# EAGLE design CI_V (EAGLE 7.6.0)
DATABASE: /Users/Kevin/working/CAD_Parts/IHC_Parts_DB.txt

## Sheet 1 of 4: CI-V Arduino Shield
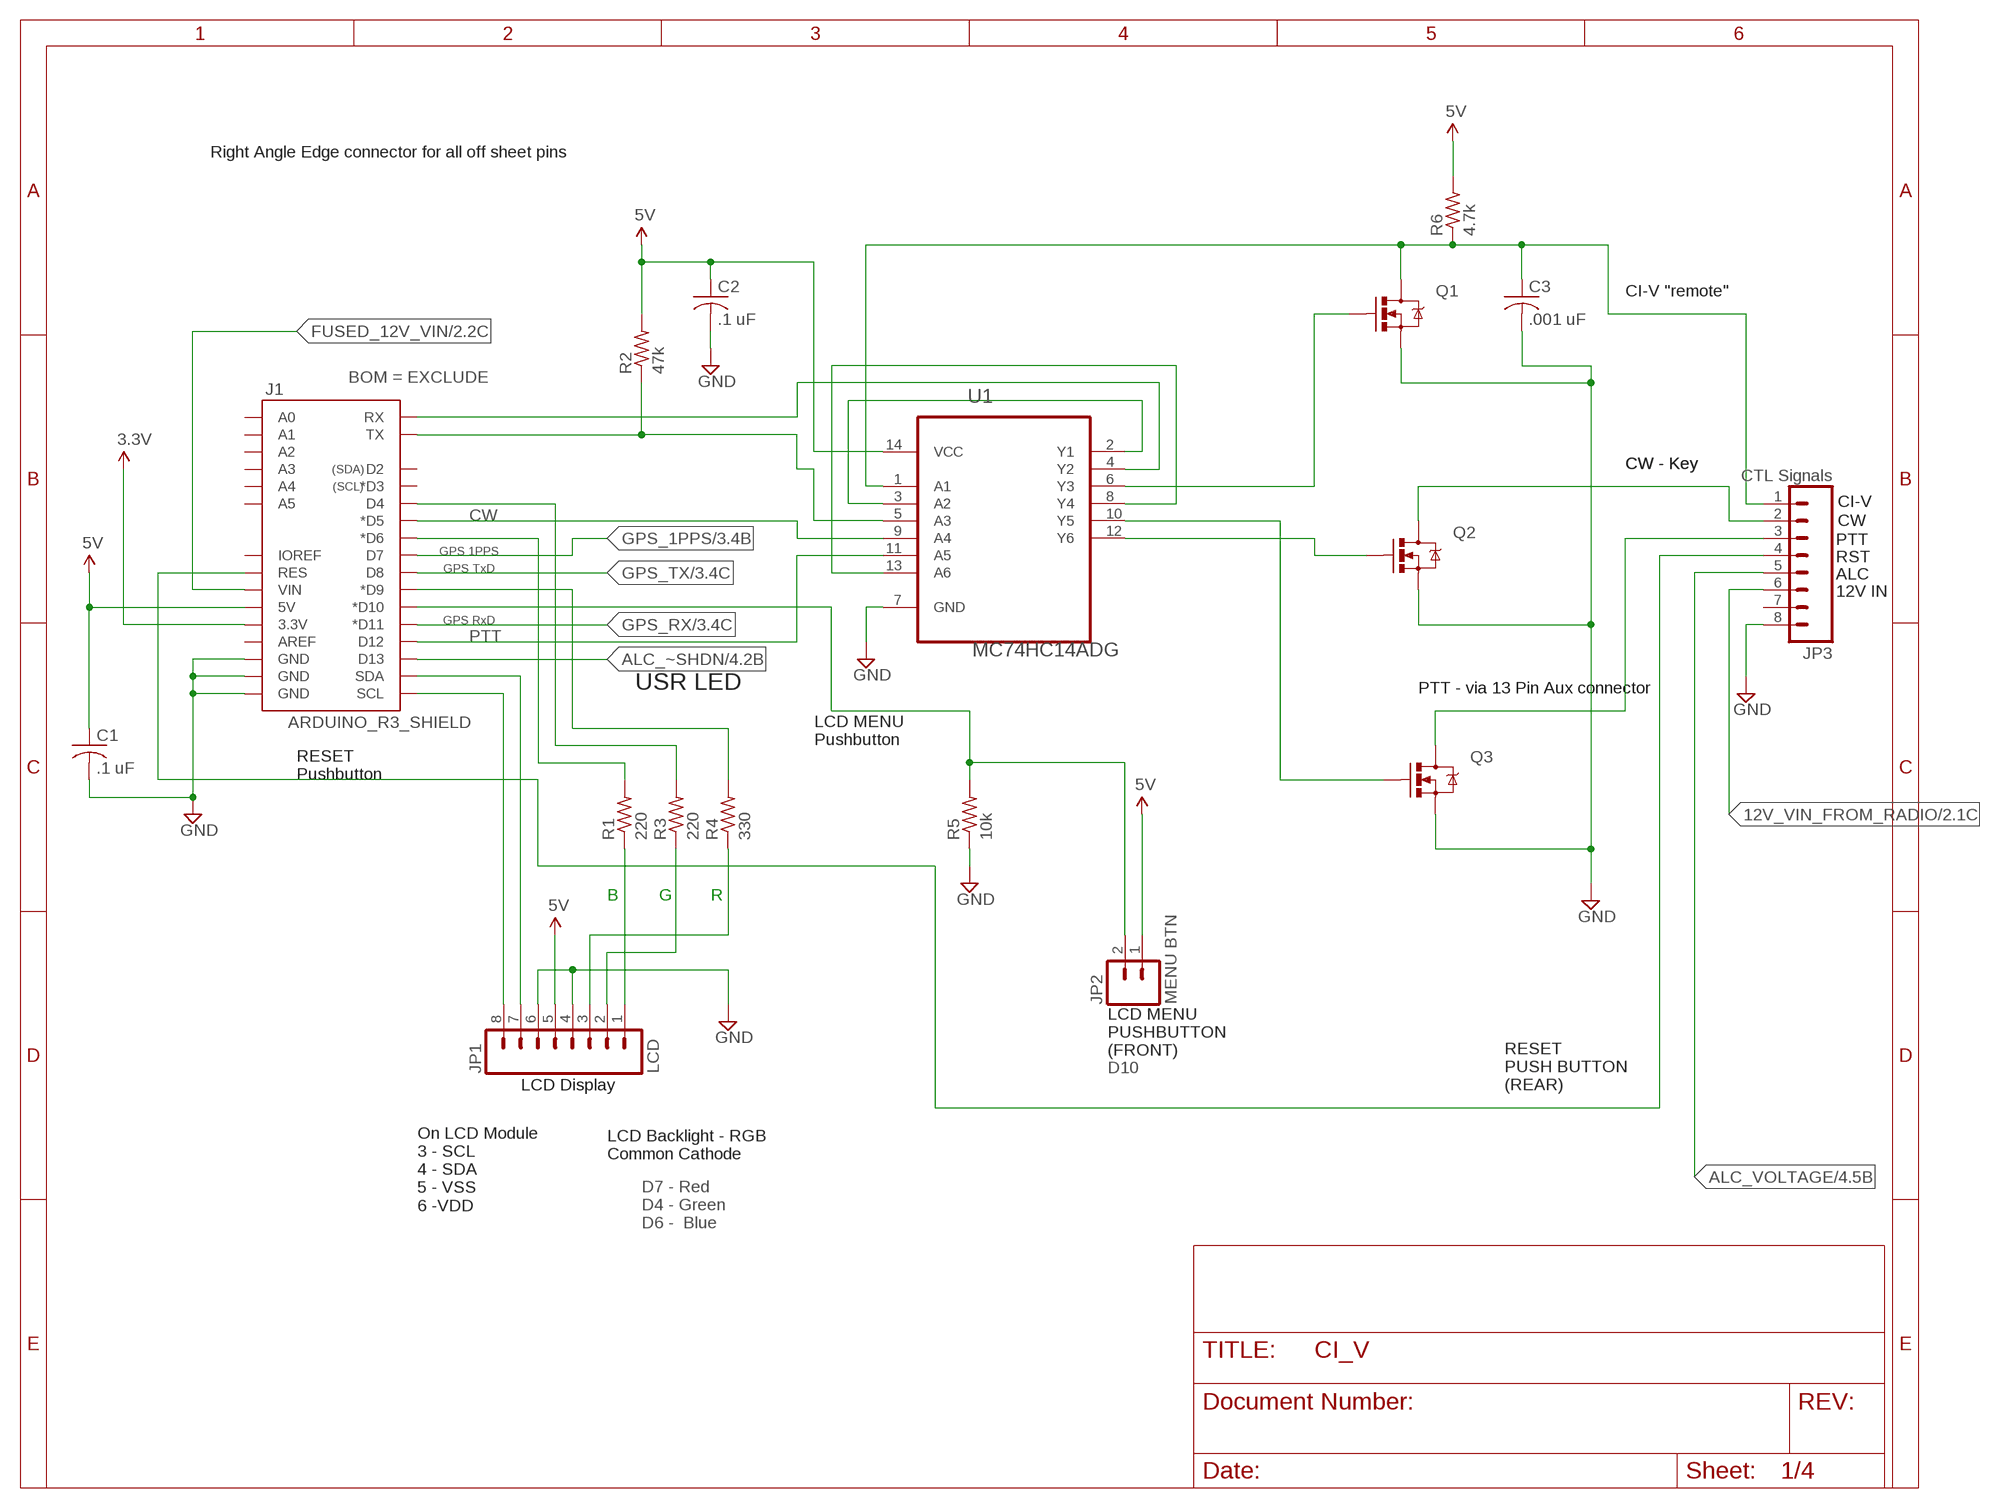
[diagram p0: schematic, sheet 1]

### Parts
C1  .1 uF  C-USC0805  [C0805]
C2  .1 uF  C-USC0805  [C0805]
C3  .001 uF  C-USC0805  [C0805]
J1  ARDUINO_R3_SHIELD  [UNO_R3_SHIELD]
JP1  LCD  M08NO_SILK  [1X08_PIN1_NO_SILK]
JP2  MENU BTN  M02PTH  [1X02]
JP3  CTL Signals  M08NO_SILK  [1X08_PIN1_NO_SILK]
Q1  MOSFET-NCHANNELBSS123LT1G  [SOT23-3]
Q2  MOSFET-NCHANNELBSS123LT1G  [SOT23-3]
Q3  MOSFET-NCHANNELBSS123LT1G  [SOT23-3]
R1  220  R-US_R0805  [R0805]
R2  47k  R-US_R0805  [R0805]
R3  220  R-US_R0805  [R0805]
R4  330  R-US_R0805  [R0805]
R5  10k  R-US_R0805  [R0805]
R6  4.7k  R-US_R0805  [R0805]
U1  MC74HC14ADG  [SOIC127P600X175-14N]

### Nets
3.3V: J1.3.3V ; also sheet 3
5V: C1.1 C2.1 J1.5V JP1.5 JP2.1 R2.2 R6.2 U1.14(VCC) ; also sheet 4
12V_VIN_FROM_RADIO: JP3.6 ; also sheet 2
ALC_VOLTAGE: JP3.5 ; also sheet 4
ALC_~SHDN: J1.D13 ; also sheet 4
CW: J1.D5(*D5) U1.9(A4)
FUSED_12V_VIN: J1.VIN ; also sheet 2
GND: C1.2 C2.2 C3.2 J1.GND@0(GND) J1.GND@1(GND) J1.GND@2(GND) JP1.4 JP1.6 JP3.8 Q1.2(S) Q2.2(S) Q3.2(S) R5.1 U1.7(GND) ; also sheet 2,3,4
GPS_1PPS: J1.D7 ; also sheet 3
GPS_RX: J1.D11(*D11) ; also sheet 3
GPS_TX: J1.D8 ; also sheet 3
HARD_RX: J1.RX U1.4(Y2)
HARD_TX: J1.TX R2.1 U1.5(A3)
N$1: C3.1 JP3.1 Q1.3(D) R6.1 U1.1(A1)
N$2: JP3.2 Q2.3(D)
N$3: JP3.3 Q3.3(D)
N$4: Q1.1(G) U1.6(Y3)
N$5: JP1.1 R1.1
N$7: JP1.2 R3.1
N$8: U1.2(Y1) U1.3(A2)
N$9: Q2.1(G) U1.12(Y6)
N$10: Q3.1(G) U1.10(Y5)
N$12: J1.SCL JP1.8
N$13: U1.8(Y4) U1.13(A6)
N$14: J1.SDA JP1.7
N$15: JP1.3 R4.1
N$16: J1.D6(*D6) R1.2
N$17: J1.D4 R3.2
N$18: J1.D9(*D9) R4.2
N$19: J1.D10(*D10) JP2.2 R5.2
N$20: J1.RES JP3.4
PTT: J1.D12 U1.11(A5)
Unconnected: J1.A0 J1.A1 J1.A2 J1.A3 J1.A4 J1.A5 J1.AREF J1.D2 J1.D3(*D3) J1.IOREF JP3.7

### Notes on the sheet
- Right Angle Edge connector for all off sheet pins
- CI-V "remote"
- CW - Key | CW - Key
- CI-V
- CW
- PTT
- GPS 1PPS
- RST
- GPS TxD
- ALC
- 12V IN
- GPS RxD
- USR LED | PTT - via 13 Pin Aux connector
- LCD MENU
  Pushbutton
- RESET
  Pushbutton
- B | G | R
- LCD MENU
  PUSHBUTTON
  (FRONT)
- D10
- LCD Display
- RESET
  PUSH BUTTON
  (REAR)
- LCD Backlight - RGB
  Common Cathode
- On LCD Module
  3 - SCL
  4 - SDA
  5 - VSS
  6 -VDD
- D7 - Red
  D4 - Green
  D6 -  Blue

## Sheet 2 of 4: Power
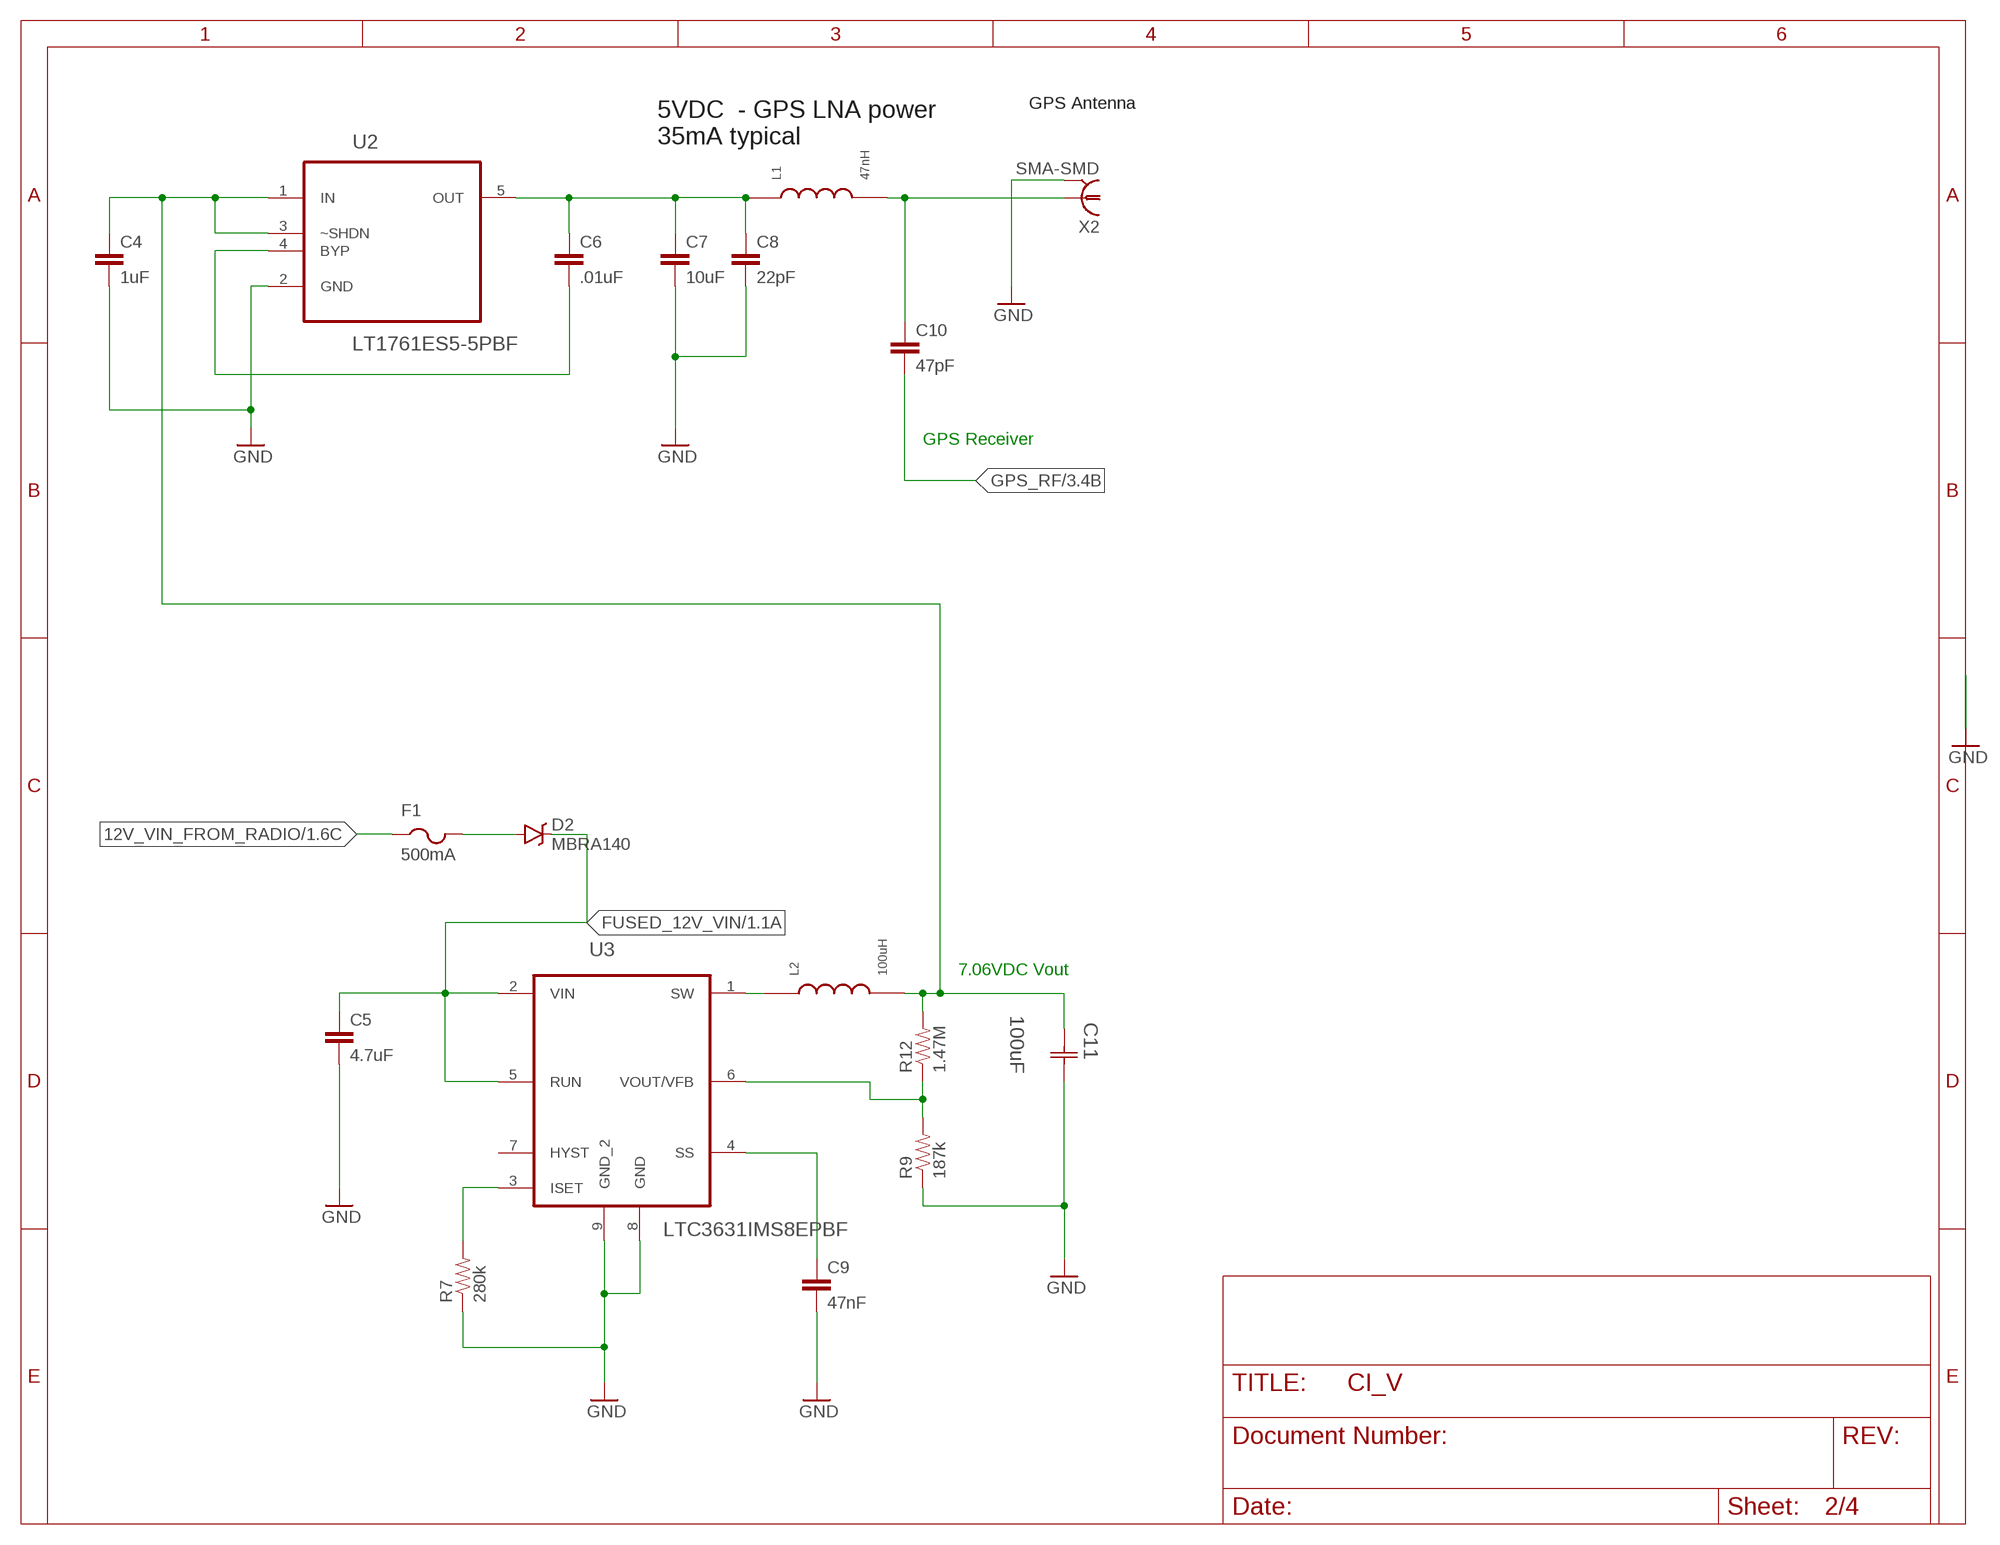
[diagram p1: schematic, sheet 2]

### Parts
C4  1uF  CAP0805  [0805]
C5  4.7uF  CAP1210  [1210]
C6  .01uF  CAP0805  [0805]
C7  10uF  CAP1210  [1210]
C8  22pF  CAP0805  [0805]
C9  47nF  CAP0805  [0805]
C10  47pF  CAP0805  [0805]
C11  100uF  THJC226K016RJN  [CAPCP6032X280N]
D2  MBRA140  DIODE-SCHOTTKY-MBRA140  [SMA-DIODE]
F1  500mA  PTCFUSE-1206  [R1206]
L1  47nH  INDUCTORMURATA  [0805]
L2  100uH  INDUCTORMURATATDK  [SLF7045]
R7  280k  RESISTOR0805-RES  [0805]
R9  187k  RESISTOR0805-RES  [0805]
R12  1.47M  RESISTOR0805-RES  [0805]
U2  LT1761ES5-5PBF  [SOT95P280X100-5N]
U3  LTC3631IMS8EPBF  [SOP65P490X110-9N]
X2  SMA-SMD  [SMA-SMD]

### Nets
7V_BUS: C4.1 C11.1(C1) L2.2 R12.2 U2.1(IN) U2.3(~SHDN)
12V_VIN_FROM_RADIO: F1.1 ; also sheet 1
FUSED_12V_VIN: C5.1 D2.C U3.2(VIN) U3.5(RUN) ; also sheet 1
GND: C4.2 C5.2 C7.2 C8.2 C9.2 C11.2(C2) R7.1 R9.1 U2.2(GND) U3.8(GND) U3.9(GND_2) X2.2@1 X2.2@2 X2.2@3 X2.2@4 X2.2@5 X2.2@6 ; also sheet 1,3,4
GPS_RF: C10.2 ; also sheet 3
ISET: R7.2 U3.3(ISET)
N$6: C10.1 L1.2 X2.1
N$21: C6.2 U2.4(BYP)
N$25: D2.A F1.2
SS: C9.1 U3.4(SS)
SW: L2.1 U3.1(SW)
VCC: C6.1 C7.1 C8.1 L1.1 U2.5(OUT)
VFB: R9.2 R12.1 U3.6(VOUT/VFB)
Unconnected: U3.7(HYST)

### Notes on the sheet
- GPS Antenna
- 5VDC  - GPS LNA power
  35mA typical
- GPS Receiver
- 7.06VDC Vout

## Sheet 3 of 4: GPS Receiver
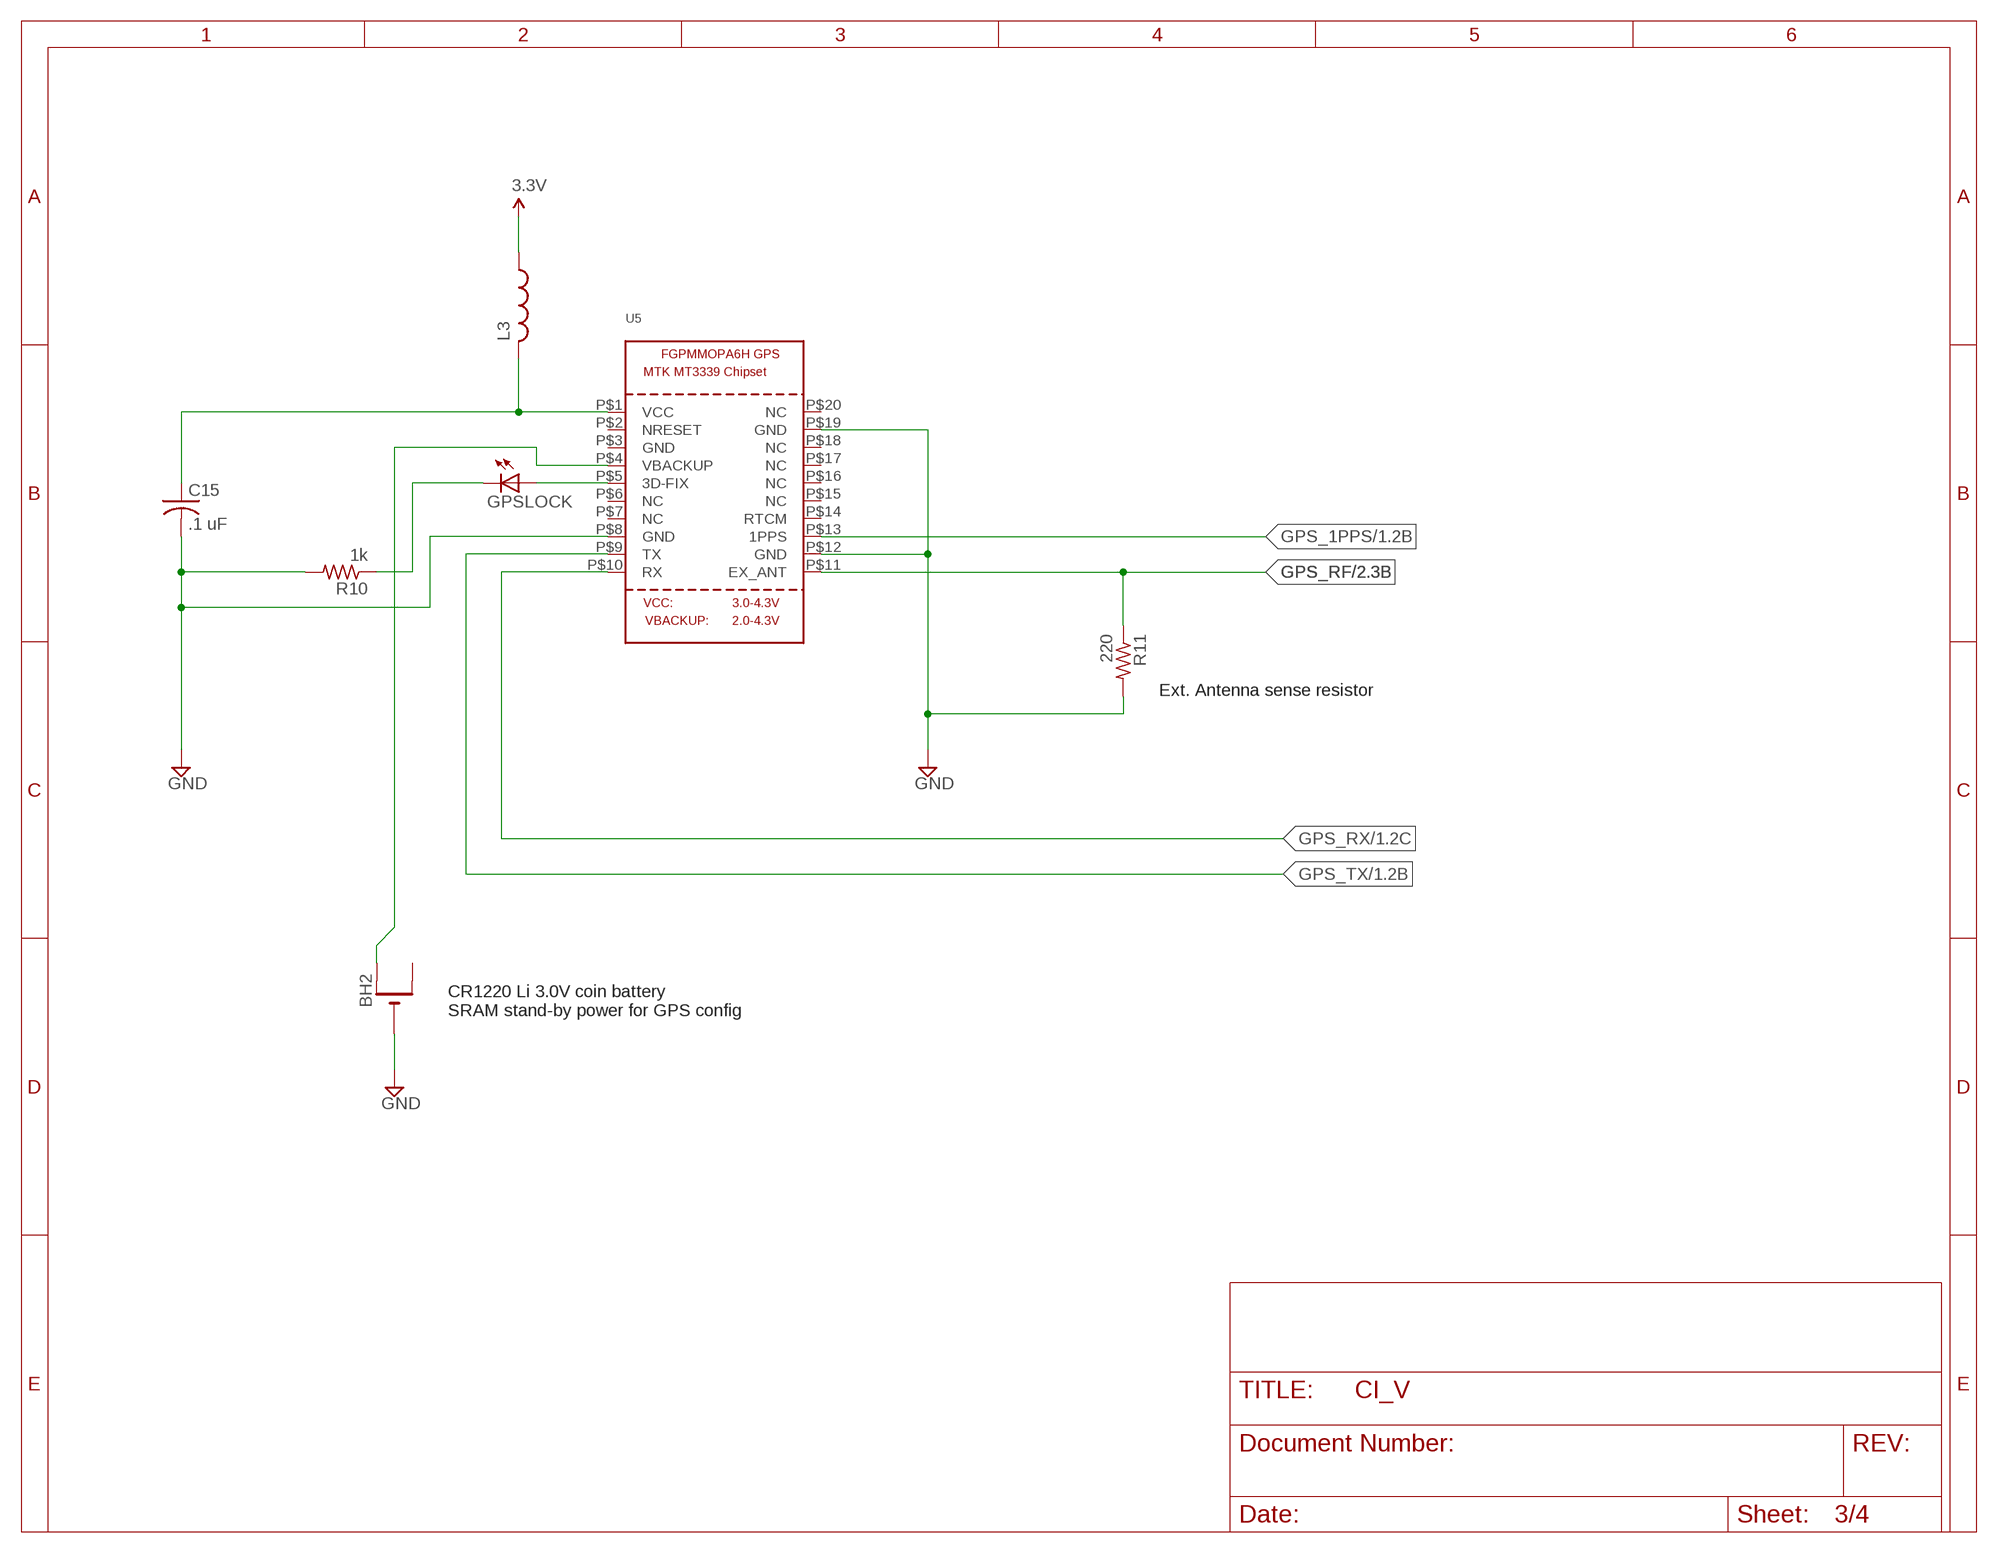
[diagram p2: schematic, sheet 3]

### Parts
BH2  CR1220SMT  [CR1220-SMD]
C15  .1 uF  C-USC0805  [C0805]
GPSLOCK  LEDCHIPLED_0805  [CHIPLED_0805]
L3  L-USL2012C  [L2012C]
R10  1k  R-US_R0805  [R0805]
R11  220  R-US_R0805  [R0805]
U5  GPS_FGPMMOPA6H  [FGPMMOPA6H]

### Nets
3.3V: L3.1 ; also sheet 1
GND: BH2.- C15.2 R10.2 R11.2 U5.P$8(GND) U5.P$12(GND) U5.P$19(GND) ; also sheet 1,2,4
GPS_1PPS: U5.P$13(1PPS) ; also sheet 1
GPS_BATT: BH2.+$1(+) U5.P$4(VBACKUP)
GPS_RF: R11.1 U5.P$11(EX_ANT) ; also sheet 2
GPS_RX: U5.P$10(RX) ; also sheet 1
GPS_TX: U5.P$9(TX) ; also sheet 1
N$11: C15.1 L3.2 U5.P$1(VCC)
N$22: GPSLOCK.A U5.P$5(3D-FIX)
N$23: GPSLOCK.C R10.1
Unconnected: BH2.+$2(+1) U5.P$2(NRESET) U5.P$3(GND) U5.P$6(NC) U5.P$7(NC) U5.P$14(RTCM) U5.P$15(NC) U5.P$16(NC) U5.P$17(NC) U5.P$18(NC) U5.P$20(NC)

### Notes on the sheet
- Ext. Antenna sense resistor
- CR1220 Li 3.0V coin battery
  SRAM stand-by power for GPS config

## Sheet 4 of 4: ALC control
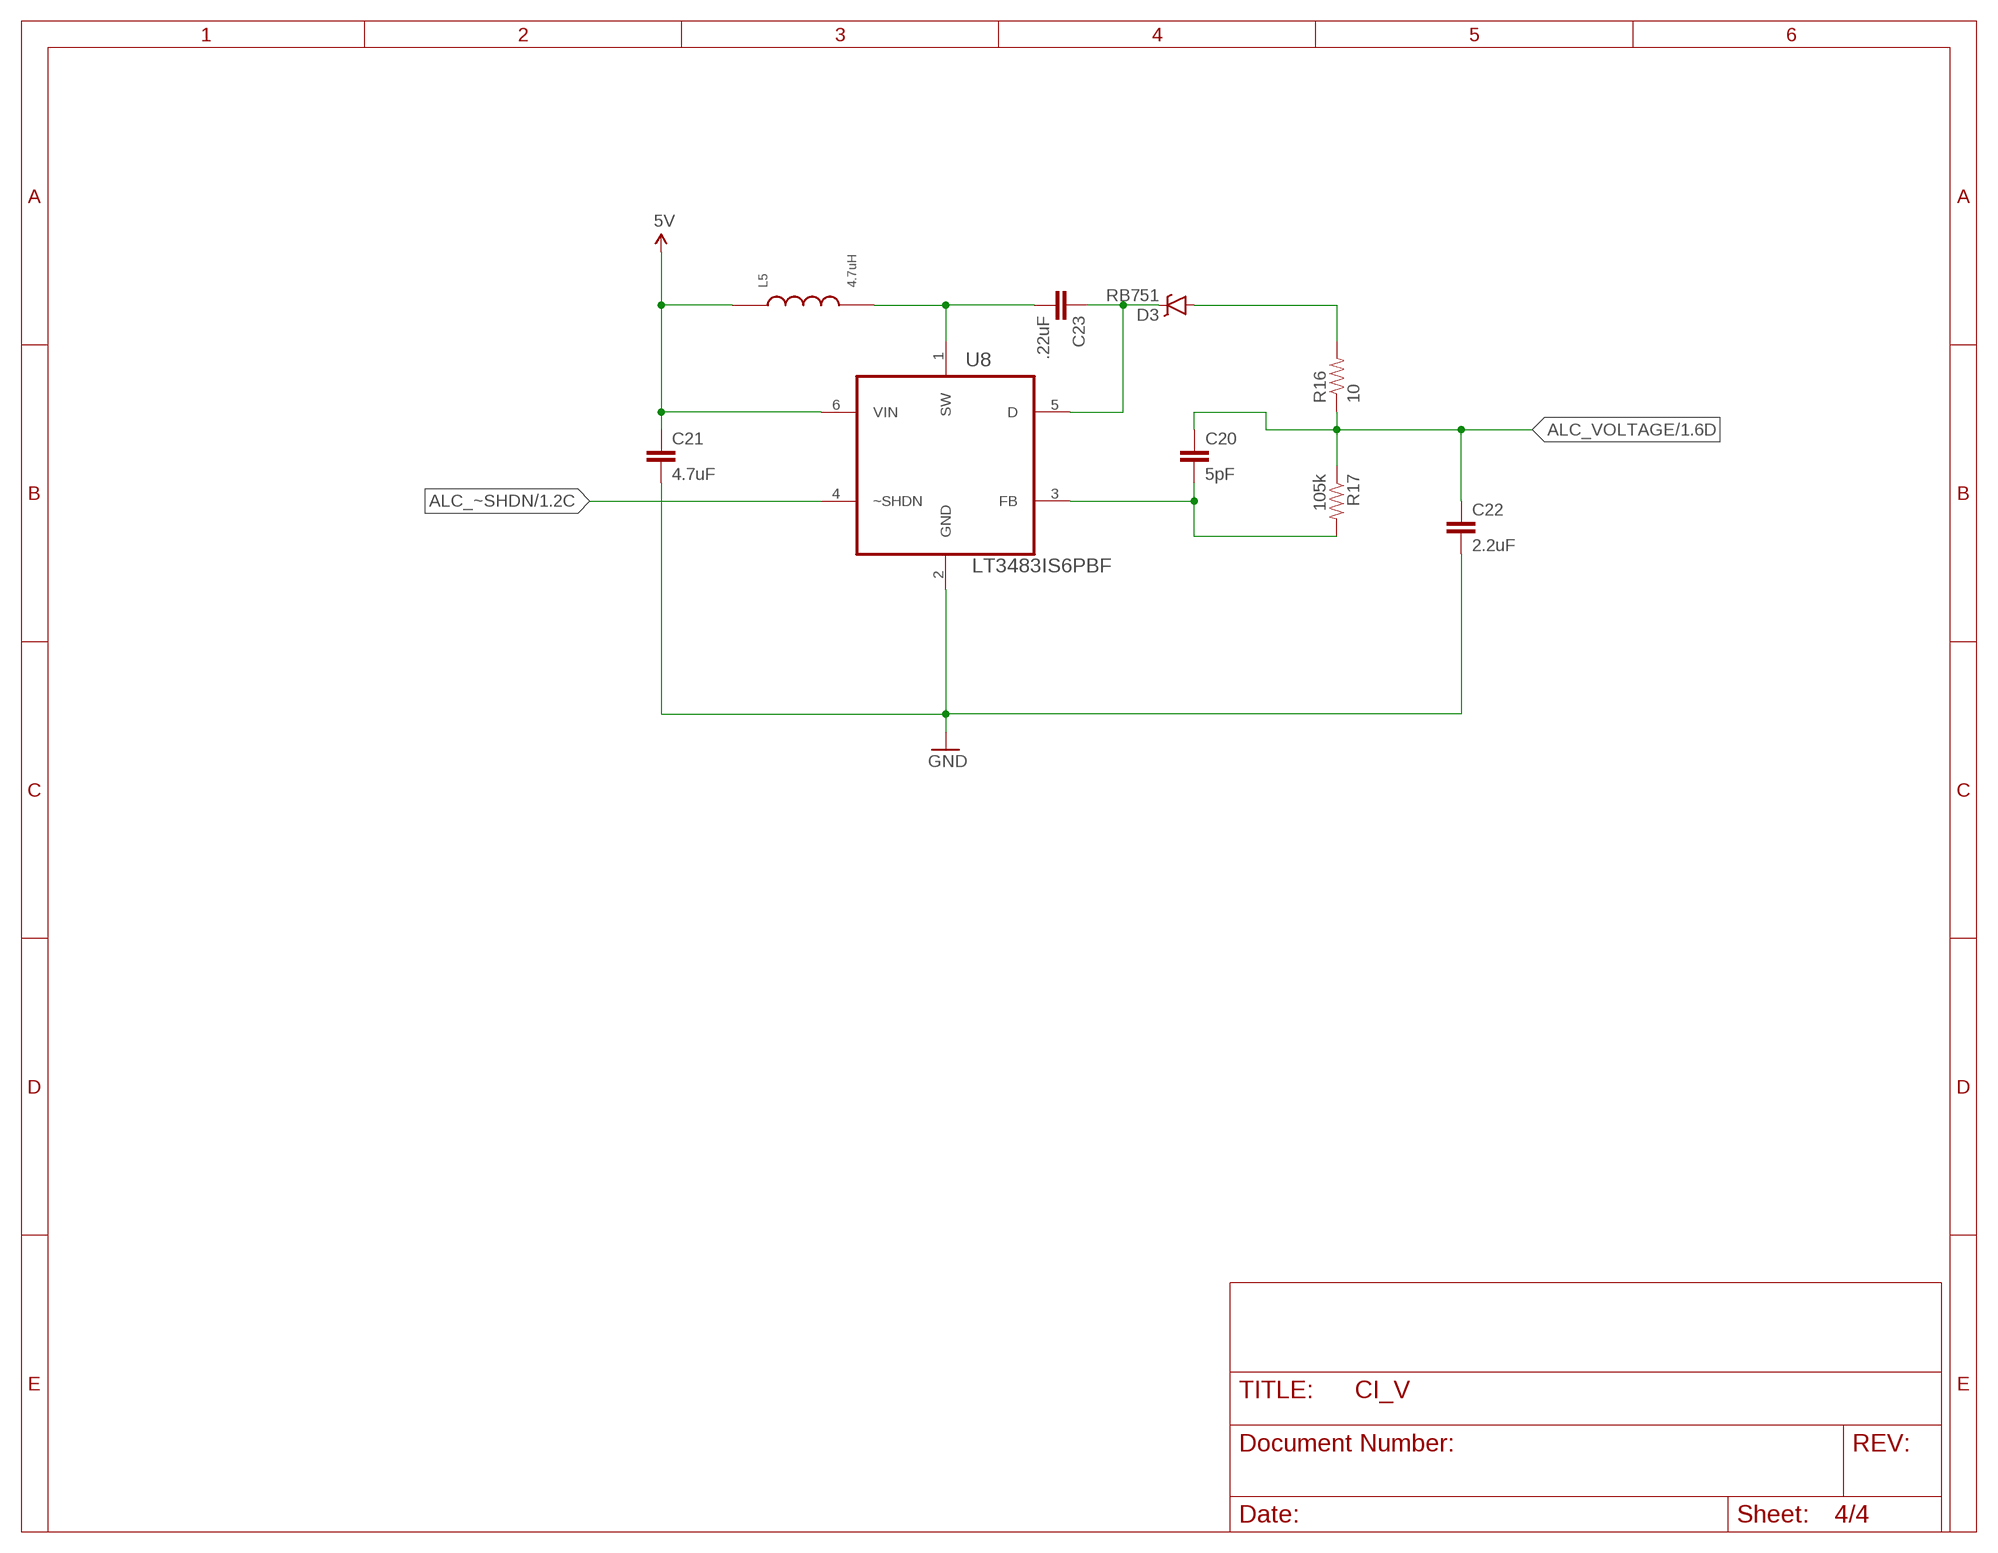
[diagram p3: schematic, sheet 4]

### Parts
C20  5pF  CAP0805  [0805]
C21  4.7uF  CAP1210  [1210]
C22  2.2uF  CAP0805  [0805]
C23  .22uF  CAP0805  [0805]
D3  RB751  DIODE-SCHOTTKY-RB751  [SOD-523]
L5  4.7uH  INDUCTORMURATA  [0805]
R16  10  RESISTOR0805-RES  [0805]
R17  105k  RESISTOR0805-RES  [0805]
U8  LT3483IS6PBF  [SOT95P280X100-6N]

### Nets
5V: C21.1 L5.1 U8.6(VIN) ; also sheet 1
ALC_VOLTAGE: C20.1 C22.1 R16.1 R17.1 ; also sheet 1
ALC_~SHDN: U8.4(~SHDN) ; also sheet 1
GND: C21.2 C22.2 U8.2(GND) ; also sheet 1,2,3
N$28: C23.2 L5.2 U8.1(SW)
N$33: C23.1 D3.C U8.5(D)
N$34: D3.A R16.2
N$37: C20.2 R17.2 U8.3(FB)

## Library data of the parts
BH2 = IHC:CR1220: CR1216/CR1220/CR1225 12mm 3V lithium coin cell Great for battery packup. Both SMT and THM holders. Note the THM package has the ground pads on both sides of the PCB so that the masks are the same - this reduces the cost; PARTNO: 165-0001-001
C1 C2 C15 = rcl:C-US: CAPACITOR, American symbol; PARTNO: 120-0001-010
C3 = rcl:C-US: CAPACITOR, American symbol; PARTNO: 120-0001-015
C4 = SparkFun-Capacitors:CAP: Capacitor; PARTNO: 120-0001-015
C5 C21 = SparkFun-Capacitors:CAP: Capacitor; PARTNO: 120-0003-011
C6 = SparkFun-Capacitors:CAP: Capacitor; PARTNO: 120-0001-020
C7 = SparkFun-Capacitors:CAP: Capacitor; PARTNO: 120-0003-010
C8 = SparkFun-Capacitors:CAP: Capacitor; PARTNO: 120-0004-011
C9 = SparkFun-Capacitors:CAP: Capacitor; PARTNO: 120-0001-013
C10 C20 = SparkFun-Capacitors:CAP: Capacitor; PARTNO: 120-0004-010
C11 = AVX_By_element14_Batch_1:THJC226K016RJN: Tantalum Capacitor , 2312; CAPACITANCETOLERANCE: ±10%; MPN: THJC226K016RJN; OC_FARNELL: 1707045; OC_NEWARK: 57P7383; PARTNO: 120-0005-050; SUPPLIER: AVX; VALUE: 22µF; VOLTAGERATING: 16V
C22 = SparkFun-Capacitors:CAP: Capacitor; PARTNO: 120-0002-011
C23 = SparkFun-Capacitors:CAP: Capacitor; PARTNO: 120-0001-022
D2 = SparkFun-DiscreteSemi:DIODE-SCHOTTKY: Schottky diodes in SFE's production catalog; PARTNO: 140-0001-001; PROD_ID: DIO-08053
D3 = SparkFun-DiscreteSemi:DIODE-SCHOTTKY: Schottky diodes in SFE's production catalog; PARTNO: 140-0002-001; PROD_ID: DIO-11018
F1 = adafruit:PTCFUSE: PTC fuses, resettable thermistors; PARTNO: 145-0001-001
GPSLOCK = adafruit:LED: LED; PARTNO: 160-0007-001
J1 = IHC:ARDUINO_R3_SHIELD: Shield form compatible with the Arduino Uno R3.; BOM: EXCLUDE
JP1 JP3 = SparkFun-Connectors:M08: Header 8 Standard 8-pin 0.1" header. Use with straight break away headers (SKU : PRT-00116), right angle break away headers (PRT-00553), swiss pins (PRT-00743), machine pins (PRT-00117), and female headers (PRT-00115).; PARTNO: 125-0019-001
JP2 = IHC:M02: Standard 2-pin 0.1" header. Use with; PARTNO: 125-0019-001
L1 = IHC:INDUCTOR; PARTNO: 155-0002-001
L2 = IHC:INDUCTOR; PARTNO: 155-0001-001
L3 = rcl:L-US: INDUCTOR, American symbol; PARTNO: 155-0004-001
L5 = IHC:INDUCTOR; PARTNO: 155-0003-001
Q1-Q3 = SparkFun-DiscreteSemi:MOSFET-NCHANNEL: Common NMOSFET Parts MFG P/NStore IDProd ID FDD8780TRANS-09984 SI7820DNTRANS-11055 FDS6630AIC-08089 2N7002PWTRANS-11151 FQP30N06L COM-10213TRANS-10060 BSS123LT1GTRANS-08345 BSS138TRANS-00830 BS170 2N7000; PARTNO: 185-0001-001; PROD_ID: TRANS-08345
R1 R3 R11 = rcl:R-US_: RESISTOR, American symbol; PARTNO: 110-0001-010
R2 R6 = rcl:R-US_: RESISTOR, American symbol; PARTNO: 110-0001-030
R4 R5 = rcl:R-US_: RESISTOR, American symbol; PARTNO: 110-0001-025
R7 = SparkFun-Passives:RESISTOR: Resistor; PARTNO: 110-0002-015
R9 = SparkFun-Passives:RESISTOR: Resistor; PARTNO: 110-0002-020
R10 = rcl:R-US_: RESISTOR, American symbol; PARTNO: 110-0001-029
R12 = SparkFun-Passives:RESISTOR: Resistor; PARTNO: 110-0002-010
R16 = SparkFun-Passives:RESISTOR: Resistor; PARTNO: 110-0001-027
R17 = SparkFun-Passives:RESISTOR: Resistor; PARTNO: 110-0003-010
U1 = ON Semiconductor_By_element14_Batch_1:MC74HC14ADG: Hex Schmitt-Trigger Inverter; MPN: MC74HC14ADG; OC_FARNELL: 9666931; OC_NEWARK: 71J5595; PACKAGE: SOIC-14; PARTNO: 200-0001-001; SUPPLIER: ON SEMICONDUCTOR
U2 = LTC_By_element14_Batch_1:LT1761ES5-5PBF: 100mA, Low Noise,LDO Micropower Regulators; MPN: LT1761ES5-5#PBF; OC_FARNELL: 1533302; OC_NEWARK: 61M3359; PACKAGE: TSOT-23-5; PARTNO: 230-0002-001; SUPPLIER: Linear Technology
U3 = IHC:LTC3631IMS8EPBF: Step-Down Converter; MPN: LTC3631IMS8E#PBF; OC_FARNELL: -; OC_NEWARK: 24R8687; PACKAGE: MSOP-8; PARTNO: 230-0003-001; SUPPLIER: Linear Technology
U5 = adafruit:GPS_FGPMMOPA6H: GPS Module - MTK MT3339 Chipset, -165dBm sensitivity, 22 channels, 10Hz, auto-select external antenna options; PARTNO: 240-0001-001
U8 = IHC:LT3483IS6PBF: Inverting Micropower DC/DC Converters with Schottky; MPN: LT3483IS6#PBF; OC_FARNELL: -; OC_NEWARK: 84R9683; PACKAGE: TSOT-23-6; SUPPLIER: Linear Technology
X2 = con-coax:SMA-SMD: SMA 50 Ohm Straight Jack Receptacle - Surface Mount; OC_FARNELL: unknown; OC_NEWARK: unknown; PARTNO: 125-0018-001

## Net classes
0 default: clearance 0.205 mm

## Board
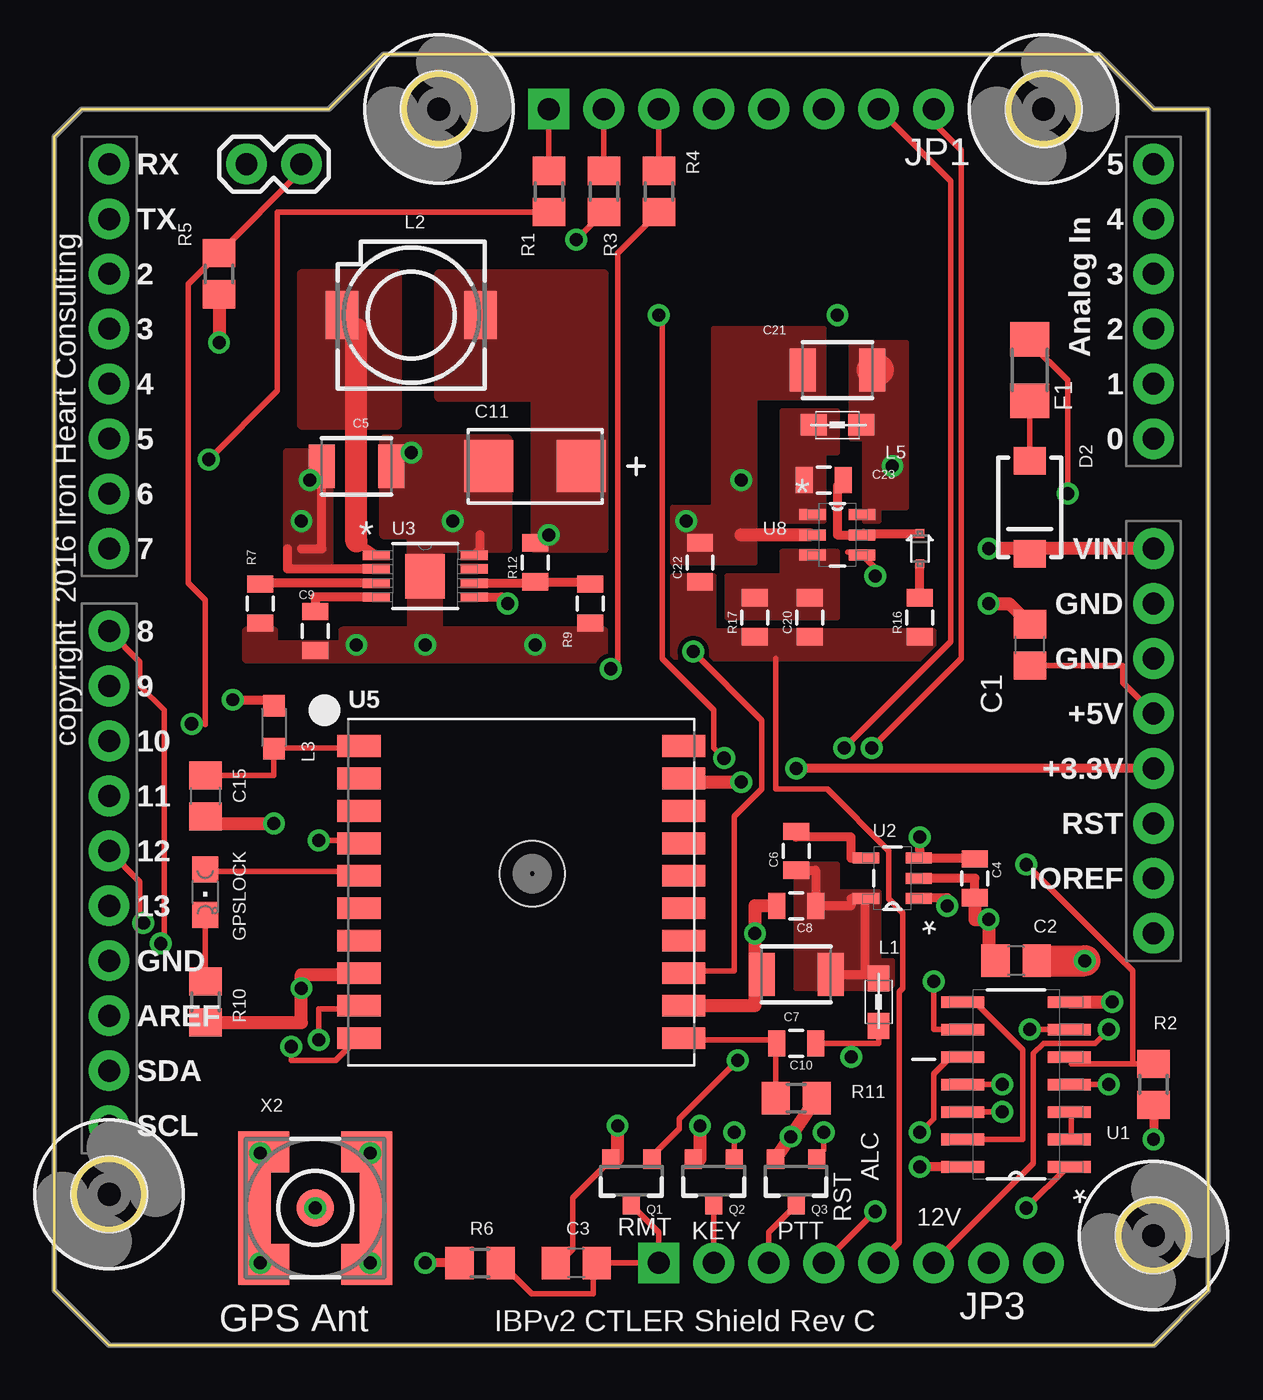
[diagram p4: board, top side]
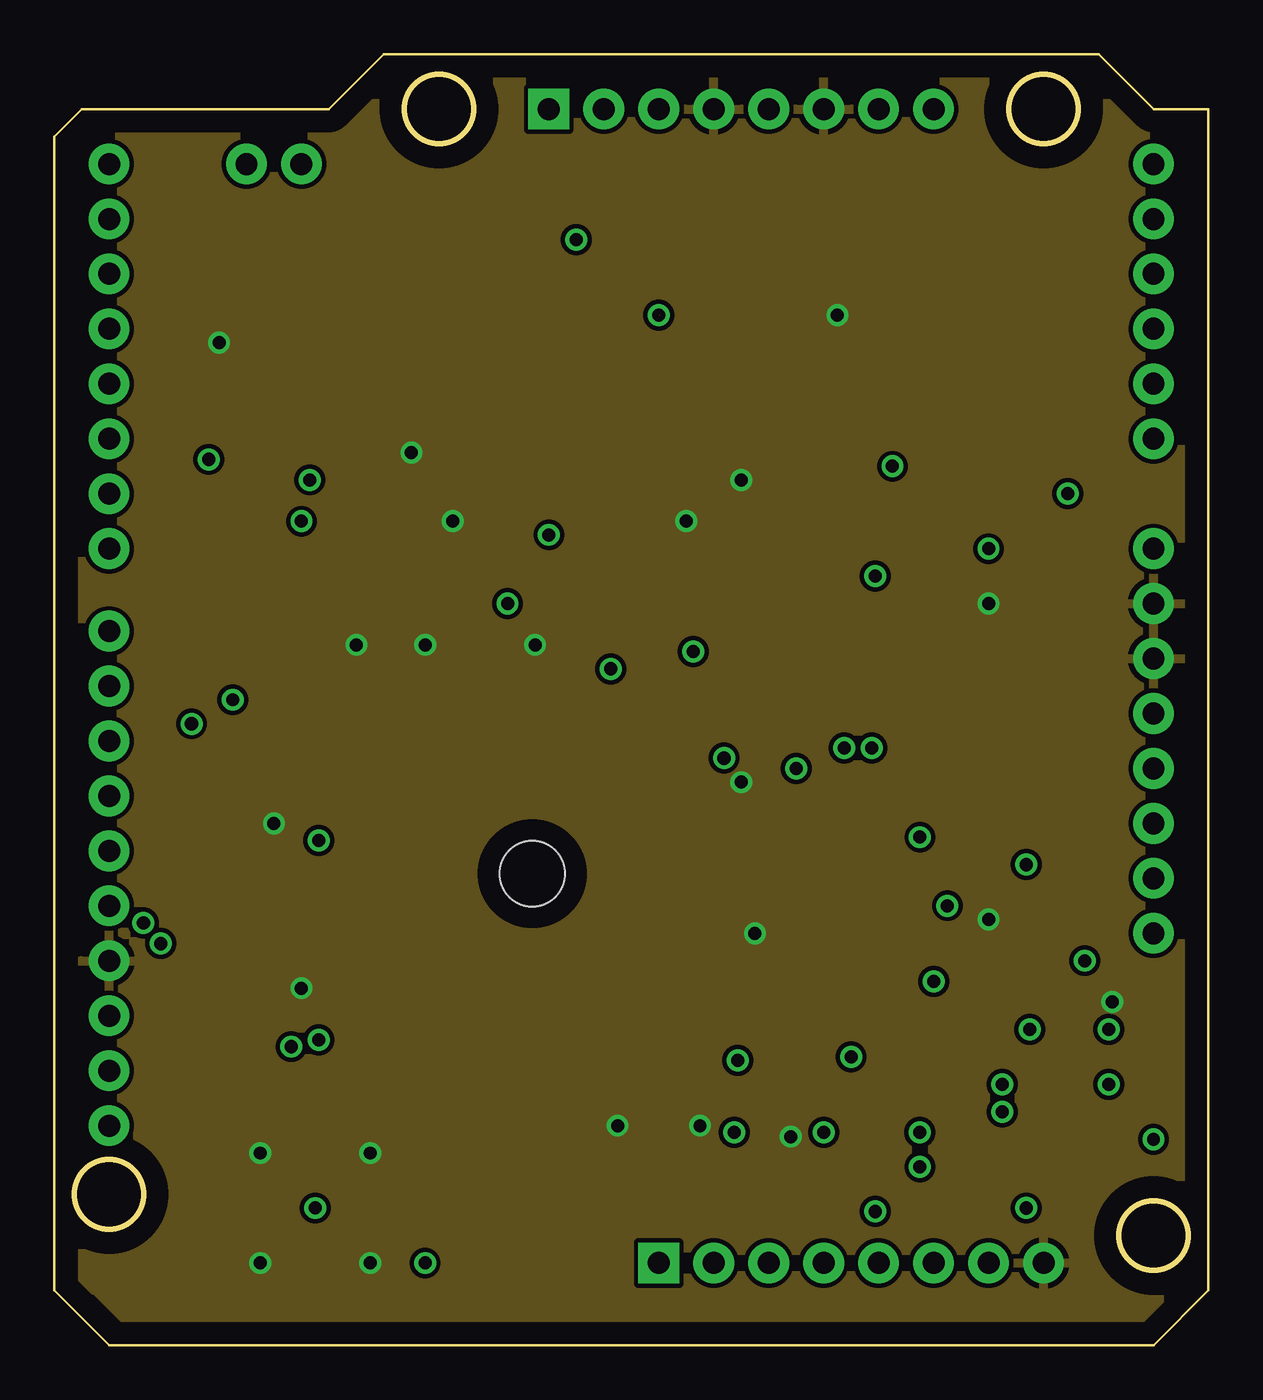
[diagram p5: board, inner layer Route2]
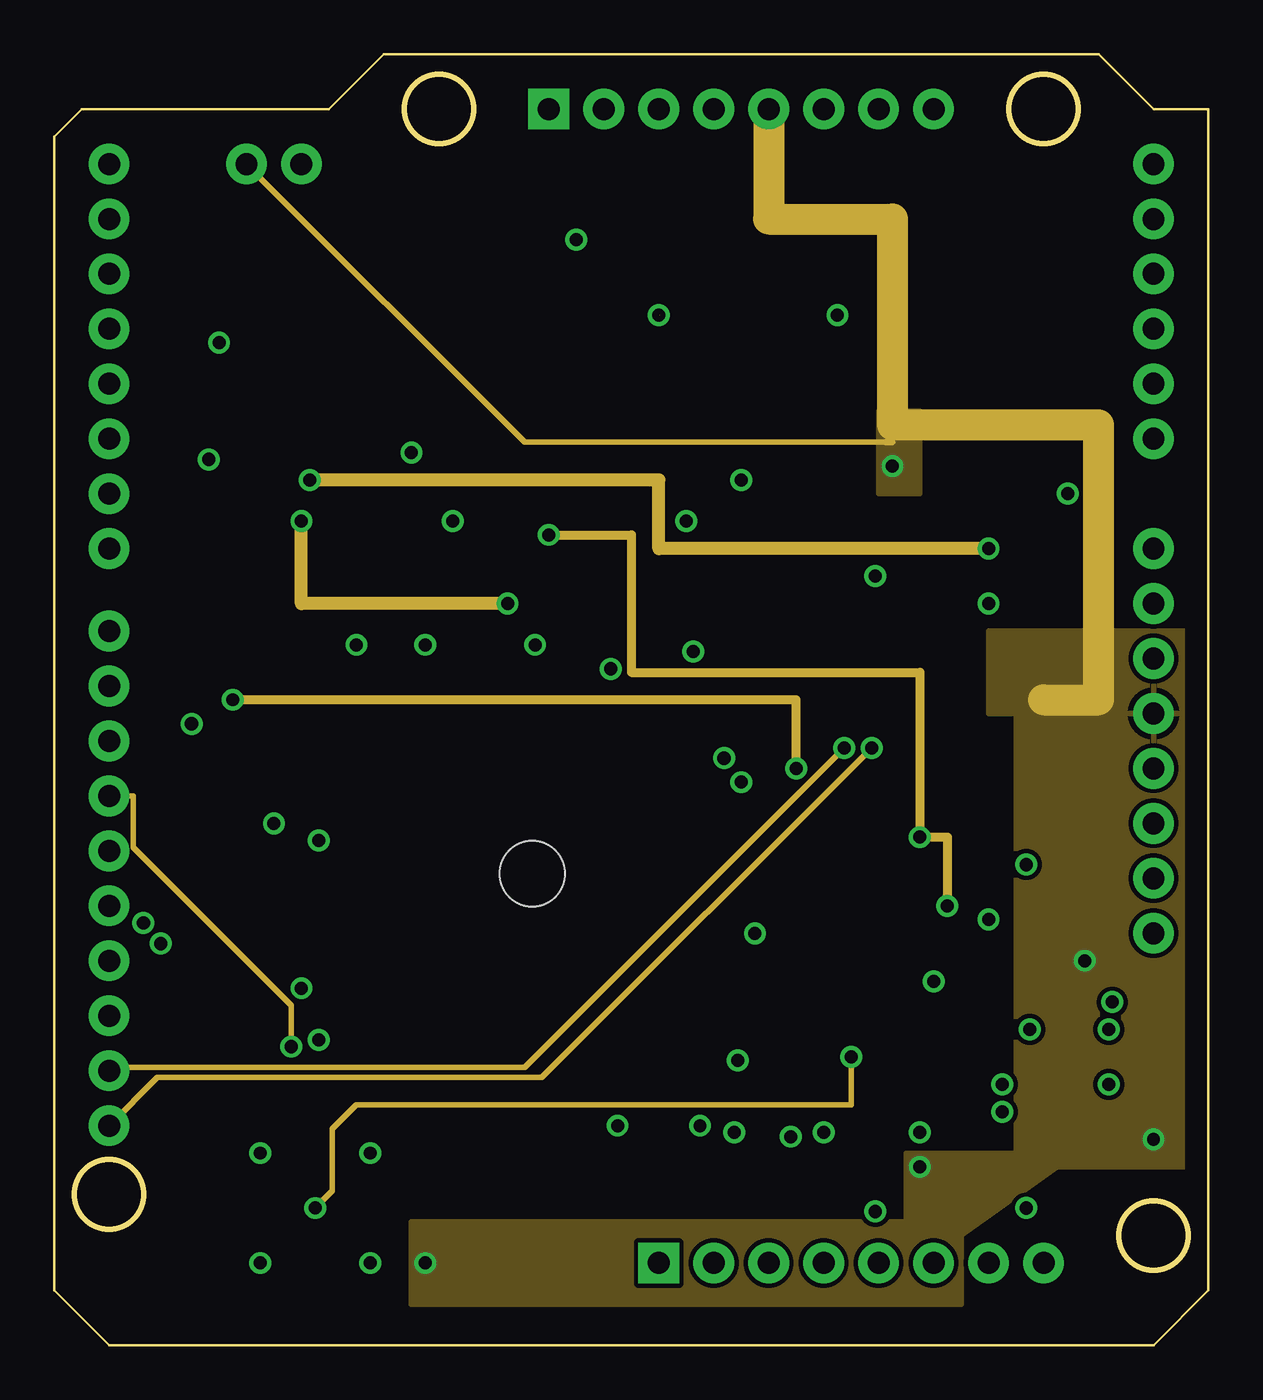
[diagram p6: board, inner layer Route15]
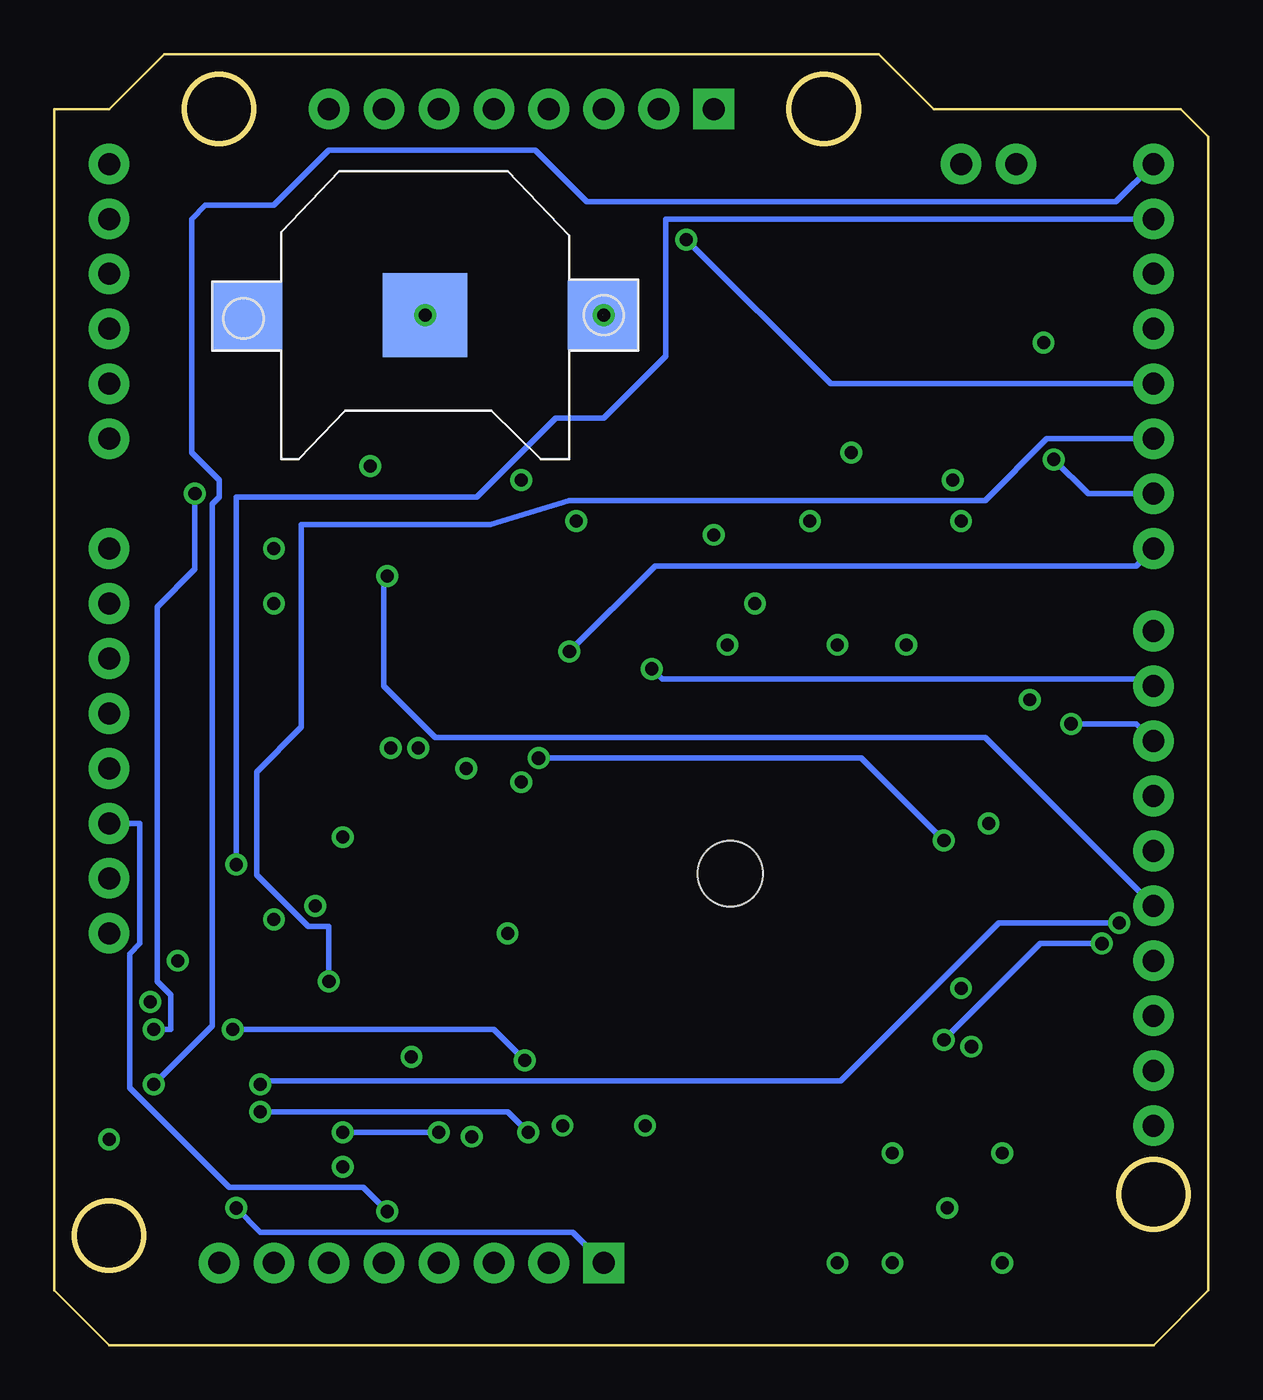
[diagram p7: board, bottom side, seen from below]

Size 53.34 x 59.69 mm. Coordinates in mm from the lower left corner, seen from the top.
Outline: circle at 45.72,57.15 radius 1.6
Outline: circle at 2.54,6.98 radius 1.6
Outline: circle at 50.8,5.08 radius 1.6
Outline: circle at 17.78,57.15 radius 1.6
Copper layers (1*2+15*16): Top 0.035mm / dielectric 0.2mm / Route2 0.035mm / dielectric 1.5mm / Route15 0.035mm / dielectric 0.2mm / Bottom 0.035mm
Design rules "default *": minimum track width 10mil, minimum drill 24mil, track to track 8mil, track to pad 8mil, pad to pad 8mil, via to via 8mil, smd to smd 8mil, copper to edge 40mil, drill to drill 8mil, minimum pad ring 10mil, minimum via ring 8mil, stop-mask expansion 4mil, vias tented up to drill 0mil, thermal gap 10mil
tRestrict: area 15.2,12.7 to 27.9,28.6

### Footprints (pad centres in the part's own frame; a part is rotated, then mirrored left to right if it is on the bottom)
CR1220-SMD = smd 3.2 x 3.2: +$1 -8.2,0; +$2 8.2,0 | smd 3.9 x 3.9: - 0,0
C0805 = smd 1.3 x 1.5: 1 -0.95,0; 2 0.95,0
0805 = smd 0.8 x 1.2: 1 -0.9,0; 2 0.9,0
1210 = smd 1.2 x 2: 1 -1.6,0; 2 1.6,0
CAPCP6032X280N = smd 2.261 x 2.413: 1 -2.134,0; 2 2.134,0
SMA-DIODE = smd 1.27 x 1.47: A -2.15,0; C 2.15,0
SOD-523 = smd 0.4 x 0.4: A -0.7,0; C 0.7,0
R1206 = smd 1.6 x 1.803: 1 -1.422,0; 2 1.422,0
CHIPLED_0805 = smd 1.2 x 1.2: A 0,-1.05; C 0,1.05
UNO_R3_SHIELD = drill 1.016 pad 1.88: 3.3V 50.8,26.67; 5V 50.8,29.21; A0 50.8,41.91; A1 50.8,44.45; A2 50.8,46.99; A3 50.8,49.53; A4 50.8,52.07; A5 50.8,54.61; AREF 2.54,15.24; D2 2.54,49.53; D3 2.54,46.99; D4 2.54,44.45; D5 2.54,41.91; D6 2.54,39.37; D7 2.54,36.83; D8 2.54,33.02; D9 2.54,30.48; D10 2.54,27.94; D11 2.54,25.4; D12 2.54,22.86; D13 2.54,20.32; GND@0 50.8,31.75; GND@1 50.8,34.29; GND@2 2.54,17.78; IOREF 50.8,21.59; NC 50.8,19.05; RES 50.8,24.13; RX 2.54,54.61; SCL 2.54,10.16; SDA 2.54,12.7; TX 2.54,52.07; VIN 50.8,36.83
1X08_PIN1_NO_SILK = drill 1.016 pad 1.88 square: 1 0,0 | drill 1.016 pad 1.88: 2 2.54,0; 3 5.08,0; 4 7.62,0; 5 10.16,0; 6 12.7,0; 7 15.24,0; 8 17.78,0
1X02 = drill 1.016 pad 1.88: 1 0,0; 2 2.54,0
0805' = smd 1.2 x 1: 1 -1.1,0; 2 1.1,0
SLF7045 = smd 1.5 x 2.2: 1 -3.2,0; 2 3.2,0
L2012C = smd 1 x 1: 1 -1,0; 2 1,0
SOT23-3 = smd 0.8 x 0.9: 1 -0.95,-1; 2 0.95,-1; 3 0,1.1
R0805 = smd 1.3 x 1.5: 1 -0.95,0; 2 0.95,0
SOIC127P600X175-14N = smd 1.981 x 0.533: 1 -2.464,3.81; 2 -2.464,2.54; 3 -2.464,1.27; 4 -2.464,0; 5 -2.464,-1.27; 6 -2.464,-2.54; 7 -2.464,-3.81; 8 2.464,-3.81; 9 2.464,-2.54; 10 2.464,-1.27; 11 2.464,0; 12 2.464,1.27; 13 2.464,2.54; 14 2.464,3.81
SOT95P280X100-5N = smd 1.219 x 0.508: 1 -1.219,0.94; 2 -1.219,0; 3 -1.219,-0.94; 4 1.219,-0.94; 5 1.219,0.94
SOP65P490X110-9N = smd 1.245 x 0.432: 1 -2.261,0.965; 2 -2.261,0.33; 3 -2.261,-0.33; 4 -2.261,-0.965; 5 2.261,-0.965; 6 2.261,-0.33; 7 2.261,0.33; 8 2.261,0.965 | smd 1.829 x 2.057: 9 0,0
FGPMMOPA6H = smd 2 x 1: P$1 -7.5,6.75; P$2 -7.5,5.25; P$3 -7.5,3.75; P$4 -7.5,2.25; P$5 -7.5,0.75; P$6 -7.5,-0.75; P$7 -7.5,-2.25; P$8 -7.5,-3.75; P$9 -7.5,-5.25; P$10 -7.5,-6.75; P$11 7.5,-6.75; P$12 7.5,-5.25; P$13 7.5,-3.75; P$14 7.5,-2.25; P$15 7.5,-0.75; P$16 7.5,0.75; P$17 7.5,2.25; P$18 7.5,3.75; P$19 7.5,5.25; P$20 7.5,6.75 | hole 3: 0.5,0.85
SOT95P280X100-6N = smd 1.219 x 0.508: 1 -1.143,0.94; 2 -1.143,0; 3 -1.143,-0.94; 4 1.143,-0.94; 5 1.143,0; 6 1.143,0.94
3,2 = hole 3.2: 0,0
SMA-SMD = smd 1.73 x 1.73: 1 0,0 | smd 2.35 x 1.9: 2@1 -2.375,2.6; 2@2 -2.375,-2.6; 2@3 2.375,-2.6; 2@4 2.375,2.6 | smd 1.5 x 3.4: 2@5 -2.8,0; 2@6 2.8,0

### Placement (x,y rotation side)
BH2  36.19,47.63 180 bottom
C1  45.08,32.38 90 top
C2  44.45,17.78 180 top
C3  24.13,3.81 180 top
C4  42.55,21.59 270 top
C5  13.97,40.64 0 top
C6  34.29,22.86 90 top
C7  34.29,17.15 180 top
C8  34.29,20.32 180 top
C9  12.06,33.02 270 top
C10  34.29,13.97 180 top
C11  22.22,40.64 180 top
C15  6.98,25.4 270 top
C20  34.92,33.66 90 top
C21  36.19,45.09 180 top
C22  29.84,36.2 90 top
C23  35.56,40.01 180 top
D2  45.08,38.74 270 top
D3  40,36.83 90 top
F1  45.08,45.09 270 top
GPSLOCK  6.98,20.95 180 top
J1  0,0 0 top
JP1  22.86,57.15 0 top
JP2  8.89,54.61 0 top
JP3  27.94,3.81 0 top
L1  47nH  [0805']  38.1,15.88 270 top
L2  16.51,47.63 0 top
L3  10.16,28.58 270 top
L5  4.7uH  [0805']  36.19,42.54 180 top
Q1  26.67,7.62 180 top
Q2  30.48,7.62 180 top
Q3  34.29,7.62 180 top
R1  22.86,53.34 270 top
R2  50.8,12.07 270 top
R3  25.4,53.34 270 top
R4  27.94,53.34 270 top
R5  7.62,49.53 90 top
R6  19.69,3.81 180 top
R7  9.52,34.29 90 top
R9  24.77,34.29 90 top
R10  6.98,15.88 270 top
R11  34.29,11.43 0 top
R12  22.22,36.2 90 top
R16  40,33.66 90 top
R17  32.38,33.66 90 top
U1  44.45,12.07 180 top
U2  38.73,21.59 180 top
U3  17.14,35.56 0 top
U5  21.59,20.95 0 top
U8  36.19,37.47 0 top
U$2  [3,2]  2.54,6.98 0 top
U$3  [3,2]  17.78,57.15 0 top
U$4  [3,2]  45.72,57.15 0 top
U$5  [3,2]  50.8,5.08 0 top
X2  12.06,6.35 0 top

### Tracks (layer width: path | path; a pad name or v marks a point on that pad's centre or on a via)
3.3V  (via drill 0.6)
  Top 0.406: J1.3.3V v34.29,26.67 | v8.25,29.84 10.16,29.84 L3.1
  Route15 0.406: v34.29,26.67 34.29,29.84 v8.25,29.84
5V  (via drill 0.6)
  Top 0.254: J1.5V 49.37,30.64 49.37,31.43 C1.1 | C2.1 45.72,17.78
  Top 0.406: U1.14 v40,8.26 | R2.2 v50.8,9.52 | R6.2 v17.14,3.81
  Top 1.422: C21.1 38.1,45.09 | 45.72,17.78 v47.62,17.78
  Route15 0.254: 38.42,41.75 21.75,41.75 JP2.1 | 38.73,41.75 38.73,42.54
  Route15 0.305: 38.42,41.75 38.73,41.75
  Route15 1.422: 45.72,29.84 48.26,29.84 48.26,42.54 38.73,42.54 38.73,52.07 33.02,52.07 JP1.5
  other vias: 38.73,40.64
  pour Top (no thermals): 37.47,38.74 37.47,41.91 36.83,41.91 36.83,46.35 39.37,46.35 39.37,38.74 38.1,38.74 38.1,38.1 37.47,38.1
  pour Route15: 16.51,5.71 39.37,5.71 39.37,8.89 44.45,8.89 44.45,29.21 43.18,29.21 43.18,33.02 52.7,33.02 52.7,8.26 46.35,8.26 41.91,5.08 41.91,1.91 16.51,1.91
  pour Route15: 40,43.18 40,39.37 38.1,39.37 38.1,43.18
7V_BUS  (via drill 0.6)
  Top 0.254: U2.1 40,20.64 40,20.7 | 40,22.86 40,22.7 U2.3
  Top 0.406: U2.3 42.55,22.53 C4.1 | 40,22.86 v40,23.5 | 40,20.7 41.27,20.7 v41.27,20.32
  Route15 0.406: v22.86,37.47 26.67,37.47 26.67,31.12 40,31.12 v40,23.5 41.27,23.5 v41.27,20.32
  pour Top (no thermals): 22.22,36.83 22.22,43.82 17.78,43.82 17.78,49.53 25.4,49.53 25.4,36.83
12V_VIN_FROM_RADIO  (via drill 0.61)
  Top 0.254: v46.83,39.37 46.83,44.61 45.08,46.35 F1.1 | v48.74,14.61 48.1,13.97 45.72,13.97 45.24,13.49 45.24,8.41 JP3.6
  Bottom 0.254: v46.83,39.37 46.83,35.88 48.58,34.13 48.58,16.83 47.94,16.19 47.94,14.61 v48.74,14.61
ALC_VOLTAGE
  Top 0.254: JP3.5 39.05,4.76 39.05,16.35 39.21,16.51 39.21,20 38.58,20.64 38.58,22.86 35.72,25.72 33.34,25.72 33.34,31.75
  pour Top (no thermals): 40.64,33.02 30.48,33.02 30.48,35.56 28.58,35.56 28.58,31.75 40.64,31.75
ALC_~SHDN  (via drill 0.61)
  Top 0.254: 36.67,36.67 37.31,36.67 U8.4 37.94,35.92 v37.94,35.56
  Bottom 0.254: J1.D13 10.32,28.1 35.72,28.1 38.1,30.48 38.1,35.4 v37.94,35.56
CW  (via drill 0.61)
  Top 0.254: U1.9 40.64,14.61 v40.64,16.83
  Bottom 0.254: v40.64,16.83 40.64,19.37 41.59,19.37 43.97,21.75 43.97,26.51 41.91,28.58 41.91,37.94 41.43,37.94 33.18,37.94 29.53,39.05 10.32,39.05 7.46,41.91 J1.D5
FUSED_12V_VIN  (via drill 0.6)
  Top 0.406: U3.2 10.8,35.89 10.8,36.83 | 11.43,36.83 12.37,36.83 C5.1 | U3.5 20.65,34.59 arc-90 v20.95,34.29
  Top 0.61: J1.VIN 45.08,36.83 D2.C 44.84,36.83 v43.18,36.83
  Route15 0.61: v20.95,34.29 11.43,34.29 v11.43,38.1 | v43.18,36.83 27.94,36.83 27.94,40.01 v11.81,40.01 11.73,40.01
  pour Top (no thermals): 12.7,41.27 12.7,36.2 10.8,36.2 10.8,41.27
GND  (via drill 0.6)
  Top 0.254: 35.08,37.47 U8.2 34.92,37.47 | 9.68,9.05 X2.2@1 | C3.2 23.34,3.81 23.97,4.45 23.97,6.83 25.56,8.41 Q1.2 | v9.52,3.81 9.68,3.81 X2.2@2 | v14.6,3.81 14.45,3.81 X2.2@3 | X2.2@4 14.45,8.89 v14.6,8.89 14.6,6.51 14.76,6.35 X2.2@6 | v9.52,8.89 9.52,6.51 9.37,6.35 X2.2@5
  Top 0.406: U3.8 19.69,36.8 19.69,37.47 | C4.2 42.55,21.59 U2.2 | v34.04,9.65 Q3.2 | X2.2@1 v9.52,8.89
  Top 0.61: 34.92,37.47 31.75,37.47 | R5.1 v7.62,46.35 | 45.41,33.66 C1.2 44.13,34.29 v43.18,34.29 | C4.2 42.55,19.69 v43.18,19.69 43.18,17.78 C2.2 | U1.7 v48.89,15.88 | C8.2 32.38,20.32 v32.38,19.05 32.38,17.15 | 32.38,17.15 C7.2 | 32.38,17.15 32.38,15.7 U5.P$12 | Q3.2 R11.2 | Q2.2 29.84,8.62 v29.84,10.16 | Q1.2 26.03,8.62 v26.03,10.16 | R10.2 11.43,14.93 v11.43,16.51 11.43,17.15 14.09,17.15 U5.P$8 | C15.2 6.98,24.13 v10.16,24.13 | U5.P$19 29.26,26.04 v31.75,26.04
  other vias: 29.21,38.1 31.75,40.01 22.22,32.38 17.14,32.38 13.97,32.38 18.41,38.1 16.51,41.27 36.19,47.63
  pour Route2: 1.27,2.54 1.27,56.52 13.33,56.52 15.88,59.05 47.62,59.05 50.16,56.52 52.7,55.88 52.7,3.18 50.8,1.27 3.17,1.27 1.9,2.54
  pour Top (no thermals): 16.51,36.2 16.51,37.47 15.24,37.47 15.24,41.91 20.95,41.91 20.95,36.83 20.32,36.83 17.78,36.83 17.78,36.2
  pour Top (no thermals): 8.89,33.02 8.89,31.75 25.4,31.75 25.4,33.02 17.78,33.02 17.78,34.93 16.51,34.93 16.51,33.02 13.33,33.02 13.33,32.38 12.7,32.38 10.16,32.38 10.16,33.02
  pour Top (no thermals): 32.38,36.2 32.38,43.82 35.56,43.82 35.56,46.99 30.48,46.99 30.48,38.74 28.58,38.74 28.58,36.2
GPS_1PPS  (via drill 0.61)
  Top 0.254: v29.53,32.07 32.7,28.89 32.7,25.72 31.43,24.45 31.43,17.3 29.21,17.3 U5.P$13
  Bottom 0.254: v29.53,32.07 25.56,36.04 3.33,36.04 J1.D7
GPS_BATT  (via drill 0.6, 0.61)  (1 unrouted)
  Top 0.254: v12.22,23.34 13.97,23.34 U5.P$4 | v30.96,27.15 30.48,27.62 30.48,29.37 28.1,31.75 28.1,47.52 BH2.+$1 v27.94,47.63
  Bottom 0.254: v12.22,23.34 16.03,27.15 v30.96,27.15
GPS_RF
  Top 0.254: 33.34,13.97 R11.1 | 33.34,13.97 33.34,14.13 29.21,14.13 U5.P$11 | 33.34,13.97 C10.2
GPS_RX  (via drill 0.61)
  Top 0.254: v10.95,13.81 10.95,13.18 13.02,13.18 13.97,14.13 U5.P$10
  Route15 0.254: v10.95,13.81 10.95,15.72 3.65,23.02 3.65,25.4 J1.D11
GPS_TX  (via drill 0.61)
  Top 0.254: v12.22,14.13 12.22,15.56 13.97,15.56 U5.P$9 | v4.92,18.57 5.08,18.73 5.08,29.37 3.97,30.48 3.97,31.59 J1.D8
  Bottom 0.254: v12.22,14.13 7.78,18.57 v4.92,18.57
HARD_RX  (via drill 0.61)
  Top 0.254: v48.74,12.07 U1.4
  Bottom 0.254: v48.74,12.07 46.04,14.76 46.04,38.89 45.72,39.21 45.72,40.01 46.99,41.27 46.99,52.07 46.35,52.71 43.18,52.71 40.64,55.24 31.11,55.24 28.73,52.86 4.29,52.86 J1.RX
HARD_TX  (via drill 0.61)
  Top 0.254: 49.85,13.02 46.99,13.02 46.99,13.34 U1.5 | 49.85,13.02 R2.1 | 49.85,13.02 49.85,17.3 v44.93,22.23
  Bottom 0.254: v44.93,22.23 44.93,39.21 33.81,39.21 30.16,42.86 27.94,42.86 25.08,45.72 25.08,52.07 J1.TX
ISET
  Top 0.406: U3.3 9.52,35.23 R7.2
N$1  (via drill 0.61)
  Top 0.254: R6.1 22.07,2.38 24.92,2.38 24.92,3.81 C3.1 JP3.1 27.94,5.24 26.67,6.51 Q1.3 | v44.93,6.35 46.83,8.26 U1.1
  Bottom 0.254: v44.93,6.35 43.81,5.24 29.37,5.24 JP3.1
N$2
  Top 0.254: JP3.2 Q2.3
N$3
  Top 0.254: JP3.3 33.02,5.24 34.29,6.51 Q3.3
N$4  (via drill 0.61)
  Top 0.254: v31.59,13.18 28.89,10.48 28.89,10 27.62,8.73 Q1.1 | U1.6 v45.08,14.61
  Bottom 0.254: v31.59,13.18 33.02,14.61 v45.08,14.61
N$5
  Top 0.254: JP1.1 R1.1
N$6  (via drill 0.6)
  Top 0.254: 36.83,13.97 38.1,13.97 L1.2 | 36.83,13.97 C10.1 | v36.83,13.34 36.83,13.97
  Route15 0.254: X2.1 12.86,7.14 12.86,10 13.97,11.11 36.51,11.11 36.83,11.11 v36.83,13.34
  other vias: 12.06,6.35
N$7
  Top 0.254: JP1.2 R3.1
N$8
  Top 0.254: U1.2 46.99,9.52 46.99,10.8 U1.3
N$9  (via drill 0.61)
  Top 0.254: v31.43,9.84 31.43,8.73 Q2.1 | U1.12 v43.81,10.8
  Bottom 0.254: v31.43,9.84 32.38,10.8 v43.81,10.8
N$10  (via drill 0.61)
  Top 0.254: v35.56,9.84 35.56,9.05 35.24,8.73 Q3.1 | v40,9.84 40.64,10.48 40.64,12.54 41.43,13.34 U1.10
  Bottom 0.254: v40,9.84 v35.56,9.84
N$11
  Top 0.254: U5.P$1 13.97,27.62 10.16,27.62 L3.2 10.16,26.35 C15.1
N$12  (via drill 0.61)
  Top 0.254: v37.78,27.62 41.91,31.75 41.91,55.24 40.64,56.52 JP1.8
  Route15 0.254: J1.SCL 4.76,12.38 22.54,12.38 v37.78,27.62
N$13
  Top 0.254: U1.13 44.77,9.52 44.77,13.65 42.55,15.88 U1.8
N$14  (via drill 0.61)
  Top 0.254: v36.51,27.62 41.43,32.54 41.43,53.82 JP1.7
  Route15 0.254: J1.SDA 2.7,12.86 21.75,12.86 v36.51,27.62
N$15
  Top 0.254: JP1.3 R4.1
N$16  (via drill 0.61)
  Top 0.254: v7.14,40.96 10.32,44.13 10.32,52.39 R1.2
  Bottom 0.254: v7.14,40.96 5.56,39.37 J1.D6
N$17  (via drill 0.61)
  Top 0.254: v24.13,51.12 R3.2
  Bottom 0.254: v24.13,51.12 17.46,44.45 J1.D4
N$18  (via drill 0.61)
  Top 0.254: v25.72,31.27 26.03,31.59 26.03,50.48 R4.2
  Bottom 0.254: v25.72,31.27 25.24,30.8 2.86,30.8 J1.D9
N$19  (via drill 0.61)
  Top 0.254: R5.2 11.43,54.29 JP2.2 | R5.2 6.19,49.05 6.19,35.24 6.98,34.45 6.98,28.7 6.95,28.73 v6.35,28.73 | R5.2
  Bottom 0.254: J1.D10 3.33,28.73 v6.35,28.73
N$20  (via drill 0.61)
  Top 0.254: v37.94,6.19 JP3.4
  Bottom 0.254: v37.94,6.19 39.05,7.3 45.24,7.3 49.85,11.91 49.85,18.1 49.37,18.57 49.37,24.13 J1.RES
N$21
  Top 0.406: U2.4 36.83,22.53 36.83,23.5 34.29,23.5 C6.2
N$22
  Top 0.254: GPSLOCK.A 6.98,21.91 13.97,21.91 13.97,21.75 U5.P$5
N$23
  Top 0.254: R10.1 GPSLOCK.C
N$25
  Top 0.254: F1.2 D2.A
N$28
  pour Top (no thermals): 35.56,38.1 33.66,38.1 33.66,43.18 36.19,43.18 36.19,41.27 35.56,41.27
N$33
  Top 0.406: C23.1 36.19,39.74 36.19,37.47 U8.5 37.4,37.53 D3.C
N$34
  Top 0.406: R16.2 D3.A
N$37
  pour Top (no thermals): 31.11,33.66 36.19,33.66 36.19,36.7 33.66,36.7 33.66,35.56 31.11,35.56
PTT  (via drill 0.61)
  Top 0.254: v43.81,12.07 U1.11 | v4.13,19.53 3.97,19.69 3.97,21.43 J1.D12
  Bottom 0.254: v43.81,12.07 43.66,12.22 16.99,12.22 9.68,19.53 v4.13,19.53
SS
  Top 0.406: U3.4 12.06,34.59 C9.1
SW
  Top 0.406: U3.1 13.97,37.16 | 13.97,46.99 13.31,46.99 L2.1
  Top 1.016: 13.97,37.16 13.97,46.99
  pour Top (no thermals): 15.88,43.82 15.88,49.53 12.06,49.53 11.43,49.53 11.43,42.54 15.88,42.54
VCC
  Top 0.406: C6.1 35.19,21.96 C8.1 36.83,20.32 36.83,20.65 U2.5 37.47,20.65 37.47,17.15 | 37.47,17.15 38.1,17.15 L1.1 | C7.1 37.47,17.15
  pour Top (no thermals): 38.73,16.51 34.29,16.51 34.29,22.23 36.19,22.23 36.19,20.95 38.1,20.95 38.1,17.78 38.73,17.78
VFB
  Top 0.406: U3.6 22.22,35.23 R12.1 24.77,35.3 R9.2

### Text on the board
tPlace: copyright 2016 Iron Heart Consulting | ALC | 12V | KEY | PTT | RST | RMT | IBPv2 CTLER Shield Rev C
tNames: GPS Ant

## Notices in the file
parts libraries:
SparkFun-Connectors: Licensing: Creative Commons ShareAlike 4.0 International - https://creativecommons.org/licenses/by-sa/4.0
